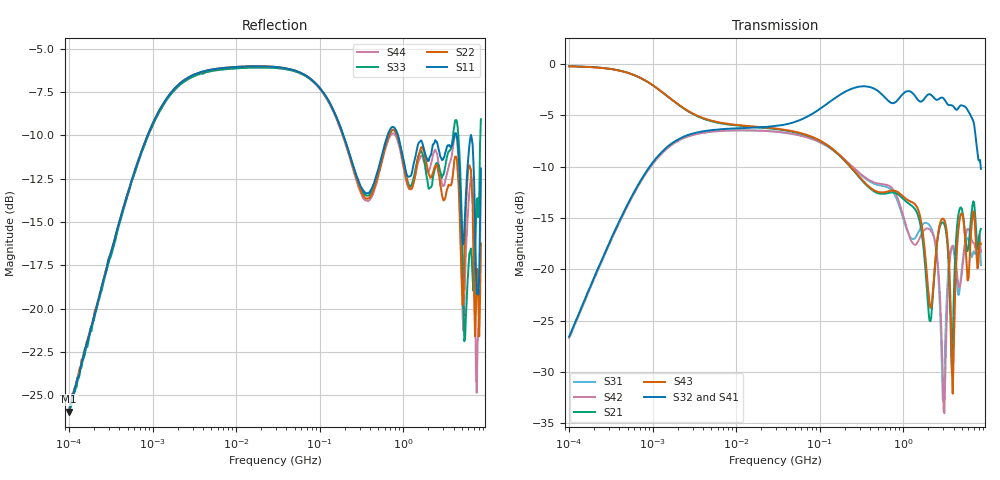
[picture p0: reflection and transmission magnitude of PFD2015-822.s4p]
# MHz S MA R 50
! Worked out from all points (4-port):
!   498 points, 100 kHz to 8.5 GHz, reference 50 ohm
!   strongest paths, dB at 100 kHz, 1.698 MHz, 29.49 MHz, 500.7 MHz, 8.5 GHz:
!     S32: -26.5, -7.7, -6.1, -2.7, -10.2
!     S41: -26.6, -7.8, -6.1, -2.7, -9.1
!     S43: -0.3, -3.5, -6.3, -12.5, -17.5
!     S21: -0.2, -3.5, -6.4, -12.6, -16.1
!     S42: -26.7, -7.9, -6.6, -11.7, -18.3
!     S31: -26.7, -7.9, -6.6, -11.8, -19.6
!   lowest |S11| = -25.9 dB at 100 kHz (marker M1), VSWR 1.11, Z = 52 + j4.74 ohm
!   |S11| at or under -10 dB: 867.1 MHz to 4.104 GHz (3.237 GHz wide, 130 % of centre); 4.353 GHz to 6.448 GHz (2.095 GHz wide, 38.8 % of centre); 6.482 GHz to end of sweep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
0.1  0.05054 64.1  0.9736 -2.8  0.04646 -96.5  0.04686 83.5
     0.9736 -2.8  0.05084 64.0  0.04705 83.8  0.04641 -96.5
     0.04646 -96.5  0.04705 83.8  0.04994 60.2  0.9712 -2.7
     0.04686 83.5  0.04641 -96.5  0.9712 -2.7  0.05129 62.4
225.1135  0.2815 -55.9  0.3194 -101.5  0.3252 78.0  0.7472 -20.1
          0.3194 -101.5  0.2789 -57.2  0.747 -20.0  0.3265 76.8
          0.3252 78.0  0.747 -20.0  0.2811 -56.0  0.3209 -101.6
          0.7472 -20.1  0.3265 76.8  0.3209 -101.6  0.276 -56.9
1306.515  0.2558 -174.8  0.2014 -106.9  0.1404 62.7  0.7043 -174.1
          0.2014 -106.9  0.2267 179.2  0.7167 -174.1  0.1338 71.0
          0.1404 62.7  0.7167 -174.1  0.2346 174.4  0.211 -106.9
          0.7043 -174.1  0.1338 71.0  0.211 -106.9  0.2294 -175.9
2713.323  0.2823 15.9  0.1583 114.0  0.07348 -9.1  0.6543 4.6
          0.1583 114.0  0.2392 -4.4  0.6772 3.4  0.08167 -2.7
          0.07348 -9.1  0.6772 3.4  0.2523 -10.0  0.1628 114.1
          0.6543 4.6  0.08167 -2.7  0.1628 114.1  0.2545 14.8
4000.492  0.3076 -136.5  0.0658 -40.8  0.1235 -94.1  0.5988 -164.5
          0.0658 -40.8  0.2533 -131.4  0.619 -167.8  0.1291 -94.3
          0.1235 -94.1  0.619 -167.8  0.3253 -144.3  0.03706 -54.5
          0.5988 -164.5  0.1291 -94.3  0.03706 -54.5  0.2994 -135.4
5383.342  0.1699 -11.8  0.1615 73.9  0.1272 88.9  0.5762 12.9
          0.1615 73.9  0.1346 -13.6  0.6217 9.3  0.1263 87.0
          0.1272 88.9  0.6217 9.3  0.08059 5.6  0.1585 65.3
          0.5762 12.9  0.1263 87.0  0.1585 65.3  0.1027 -19.2
8500  0.2539 -5.8  0.1572 39.2  0.1049 14.4  0.3518 -37.2
      0.1572 39.2  0.1543 -15.7  0.3081 -49.9  0.1214 -2.9
      0.1049 14.4  0.3081 -49.9  0.3521 -41.5  0.133 34.8
      0.3518 -37.2  0.1214 -2.9  0.133 34.8  0.2482 1.1
